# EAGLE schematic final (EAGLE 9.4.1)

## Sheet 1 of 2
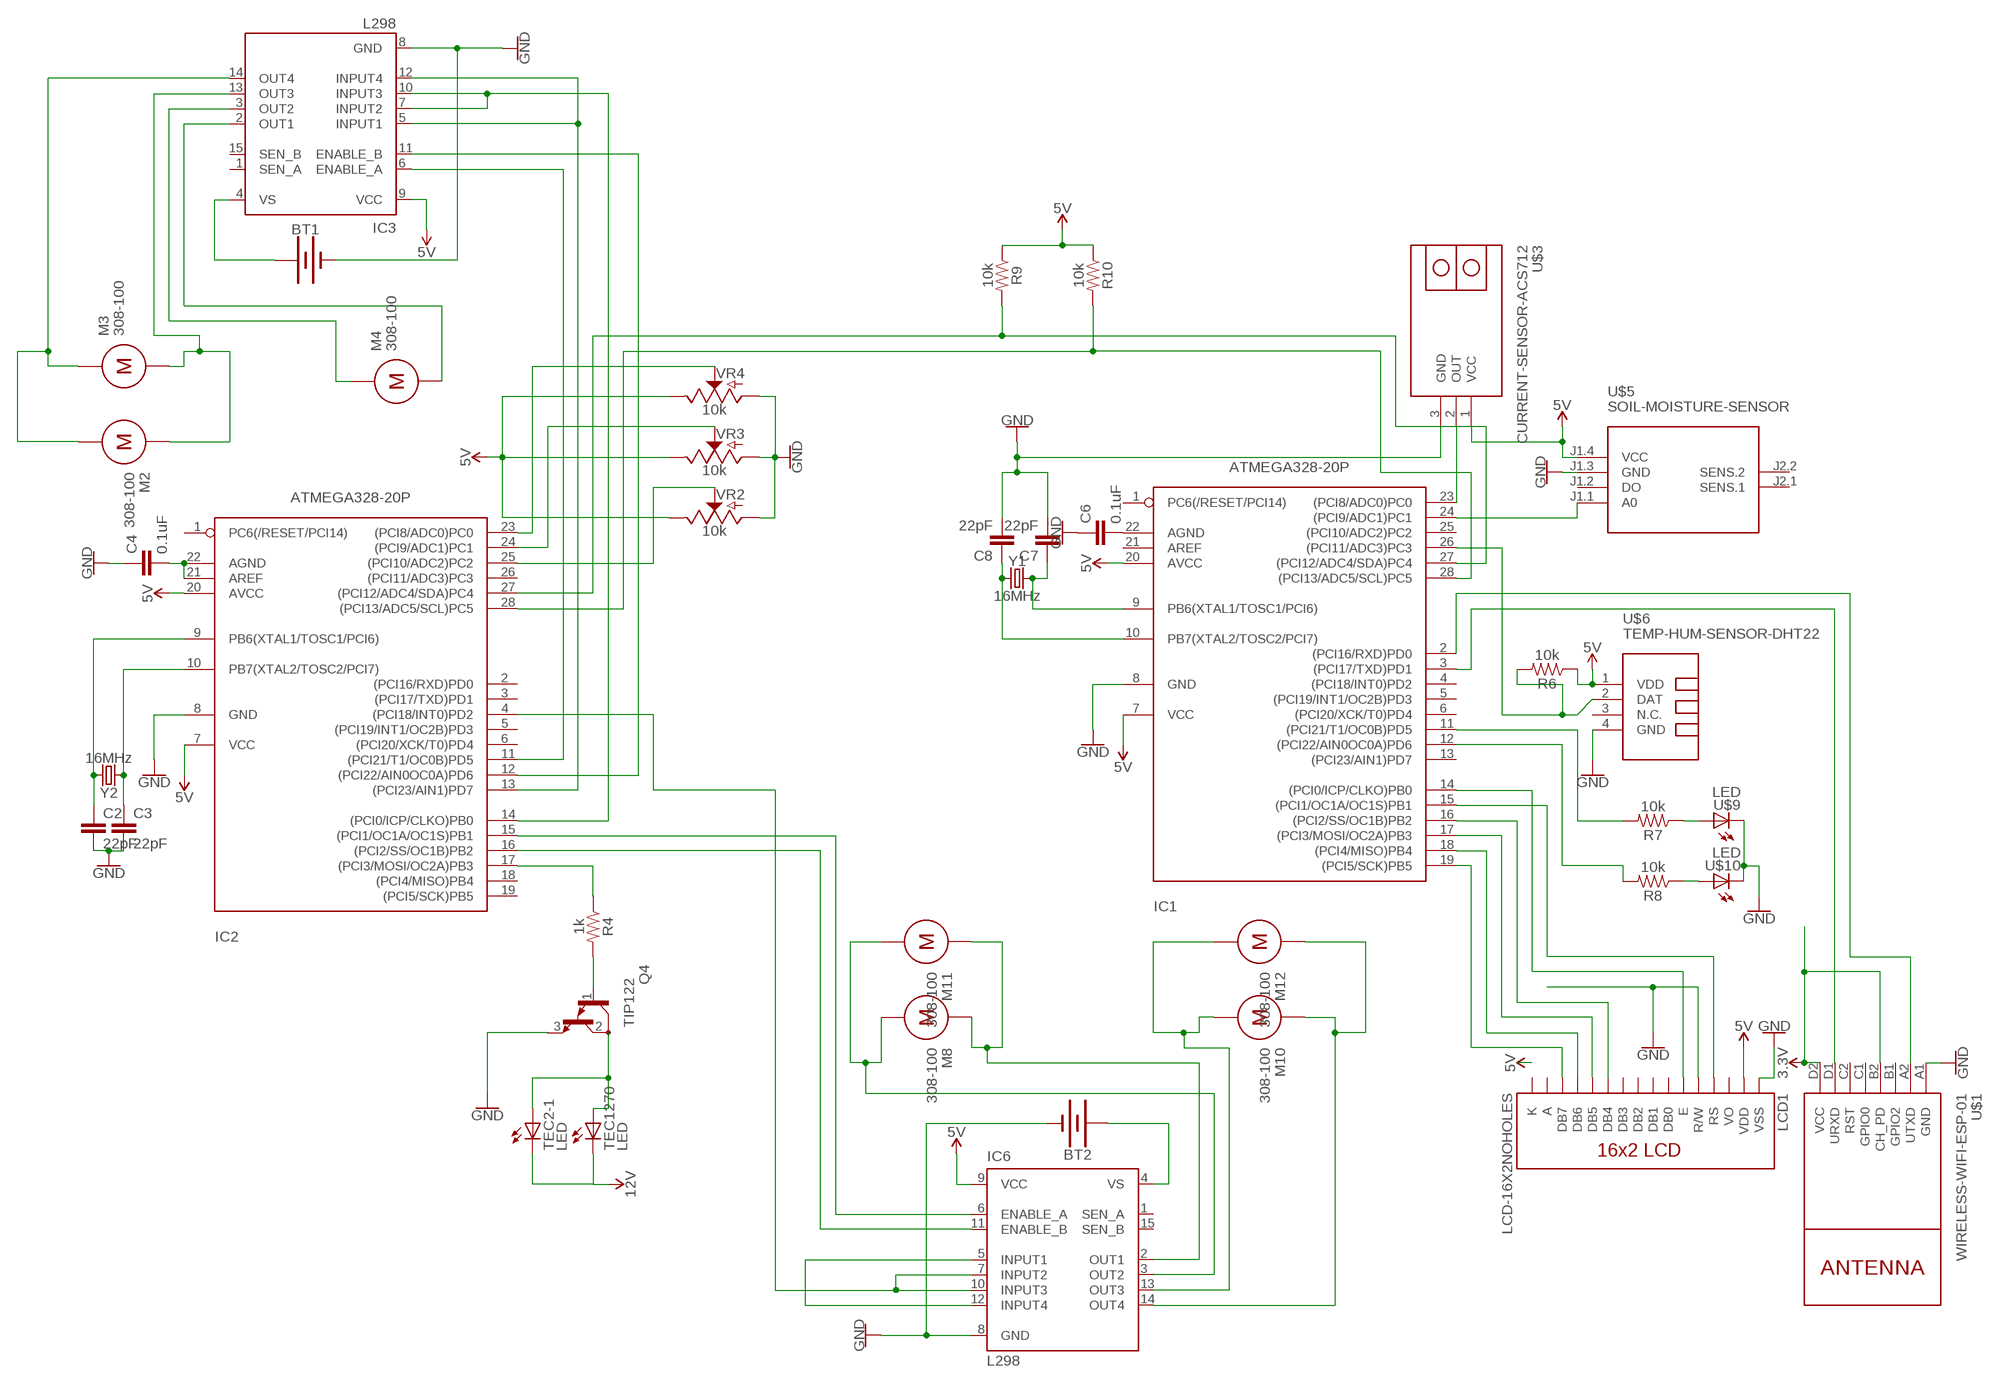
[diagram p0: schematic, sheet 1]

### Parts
BT1  BATTERY-12MM_PTH  [BATTCON_12MM_PTH]
BT2  BATTERY-12MM_PTH  [BATTCON_12MM_PTH]
C2  22pF  22PF-0603-50V-5%  [0603]
C3  22pF  22PF-0603-50V-5%  [0603]
C4  0.1uF  0.1UF-0402-16V-10%  [0402]
C6  0.1uF  0.1UF-0402-16V-10%  [0402]
C7  22pF  22PF-0603-50V-5%  [0603]
C8  22pF  22PF-0603-50V-5%  [0603]
IC1  ATMEGA328-20P  [DIL28-3]
IC2  ATMEGA328-20P  [DIL28-3]
IC3  L298  [MULTIWATT-15]
IC6  L298  [MULTIWATT-15]
LCD1  LCD-16X2NOHOLES  [LCD-16X2_NOHOLESNOSILK]
M2  308-100  [308-100]
M3  308-100  [308-100]
M4  308-100  [308-100]
M8  308-100  [308-100]
M10  308-100  [308-100]
M11  308-100  [308-100]
M12  308-100  [308-100]
Q4  TIP122  [TO220]
R4  1k  10KOHM-0603-1/10W-1%  [0603]
R6  10k  10KOHM-0603-1/10W-1%  [0603]
R7  10k  10KOHM-0603-1/10W-1%  [0603]
R8  10k  10KOHM-0603-1/10W-1%  [0603]
R9  10k  10KOHM-0603-1/10W-1%  [0603]
R10  10k  10KOHM-0603-1/10W-1%  [0603]
TEC2-1  LED  [HLMP-1790]
TEC1270  LED  [HLMP-1790]
U$1  WIRELESS-WIFI-ESP-01  [WIRELESS-WIFI-ESP-01]
U$3  CURRENT-SENSOR-ACS712  [CURRENT-SENSOR-ACS712]
U$5  SOIL-MOISTURE-SENSOR  [SOIL-MOISTURE-SENSOR]
U$6  TEMP-HUM-SENSOR-DHT22  [TEMP-HUM-SENSOR-DHT22]
U$9  LED  [HLMP-1790]
U$10  LED  [HLMP-1790]
VR2  10k  POTENTIOMETER-PTH-9MM-1/20W-20%-KIT  [POT-PTH-ALPS-KIT]
VR3  10k  POTENTIOMETER-PTH-9MM-1/20W-20%-KIT  [POT-PTH-ALPS-KIT]
VR4  10k  POTENTIOMETER-PTH-9MM-1/20W-20%-KIT  [POT-PTH-ALPS-KIT]
Y1  16MHz  CRYSTAL-16MHZPTH-HC49US  [HC49US]
Y2  16MHz  CRYSTAL-16MHZPTH-HC49US  [HC49US]

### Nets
3.3V: U$1.B2(CH_PD) U$1.D2(VCC) ; also sheet 2
5V: IC1.7(VCC) IC1.20(AVCC) IC2.7(VCC) IC2.20(AVCC) IC3.9(VCC) IC6.9(VCC) LCD1.2(VDD) R6.1 R9.1 R10.1 TEC2-1.C TEC1270.C U$3.1(VCC) U$5.J1.4(VCC) U$6.1(VDD) VR2.P$1(E) VR3.P$1(E) VR4.P$1(E) ; supply symbol labelled 12V ; also sheet 2
GND: BT1.GND(-) BT2.GND(-) C2.2 C3.2 C4.1 C6.1 C7.2 C8.2 IC1.8(GND) IC2.8(GND) IC3.8(GND) IC6.8(GND) LCD1.1(VSS) LCD1.5(R/W) Q4.3(E) U$1.A1(GND) U$3.3(GND) U$5.J1.3(GND) U$6.4(GND) U$9.C U$10.C VR2.P$3(A) VR3.P$3(A) VR4.P$3(A) ; also sheet 2
N$1: LCD1.14(DB7)
N$2: IC1.27((PCI12/ADC4/SDA)PC4) IC2.27((PCI12/ADC4/SDA)PC4) R9.2
N$3: IC2.25((PCI10/ADC2)PC2) VR2.P$2(S)
N$4: LCD1.13(DB6)
N$5: LCD1.12(DB5)
N$7: IC1.26((PCI11/ADC3)PC3) R6.2 U$6.2(DAT)
N$8: BT2.VCC@1(+) IC6.4(VS)
N$9: IC1.2((PCI16/RXD)PD0)
N$10: IC2.23((PCI8/ADC0)PC0) VR4.P$2(S)
N$11: C4.2 IC2.21(AREF) IC2.22(AGND)
N$14: IC1.23((PCI8/ADC0)PC0) U$3.2(OUT)
N$15: IC1.24((PCI9/ADC1)PC1) U$5.J1.1(A0)
N$16: IC1.19((PCI5/SCK)PB5)
N$17: IC1.18((PCI4/MISO)PB4)
N$18: IC1.17((PCI3/MOSI/OC2A)PB3)
N$19: IC6.5(INPUT1) IC6.12(INPUT4)
N$20: IC1.16((PCI2/SS/OC1B)PB2)
N$21: IC1.14((PCI0/ICP/CLKO)PB0)
N$22: IC1.15((PCI1/OC1A/OC1S)PB1)
N$23: IC2.4((PCI18/INT0)PD2) IC6.7(INPUT2) IC6.10(INPUT3)
N$24: IC2.12((PCI22/AIN0OC0A)PD6) IC3.11(ENABLE_B)
N$25: IC2.14((PCI0/ICP/CLKO)PB0) IC3.7(INPUT2) IC3.10(INPUT3)
N$26: IC3.2(OUT1) M4.NEG
N$29: BT1.VCC@1(+) IC3.4(VS)
N$30: IC2.11((PCI21/T1/OC0B)PD5) IC3.6(ENABLE_A)
N$31: IC2.15((PCI1/OC1A/OC1S)PB1) IC6.6(ENABLE_A)
N$32: IC2.16((PCI2/SS/OC1B)PB2) IC6.11(ENABLE_B)
N$33: IC6.2(OUT1) M8.POS M11.POS
N$34: IC3.3(OUT2) M4.POS
N$35: IC6.3(OUT2) M8.NEG M11.NEG
N$36: Q4.2(C) TEC2-1.A TEC1270.A
N$38: Q4.1(B) R4.2
N$39: LCD1.11(DB4)
N$40: LCD1.6(E)
N$41: IC2.24((PCI9/ADC1)PC1) VR3.P$2(S)
N$42: IC2.17((PCI3/MOSI/OC2A)PB3) R4.1
N$43: C3.1 IC2.10(PB7(XTAL2/TOSC2/PCI7)) Y2.1
N$44: IC2.13((PCI23/AIN1)PD7) IC3.5(INPUT1) IC3.12(INPUT4)
N$45: C2.1 IC2.9(PB6(XTAL1/TOSC1/PCI6)) Y2.2
N$46: IC1.3((PCI17/TXD)PD1)
N$47: IC1.11((PCI21/T1/OC0B)PD5) R7.2
N$48: IC1.12((PCI22/AIN0OC0A)PD6) R8.2
N$49: R7.1 U$9.A
N$50: R8.1 U$10.A
N$51: C6.2 IC1.22(AGND)
N$53: LCD1.4(RS)
N$54: U$1.A2(UTXD)
N$55: U$1.D1(URXD)
N$62: C8.1 IC1.10(PB7(XTAL2/TOSC2/PCI7)) Y1.1
N$63: C7.1 IC1.9(PB6(XTAL1/TOSC1/PCI6)) Y1.2
N$92: IC1.28((PCI13/ADC5/SCL)PC5) IC2.28((PCI13/ADC5/SCL)PC5) R10.2
O1: IC6.13(OUT3) M10.NEG M12.NEG
O2: IC6.14(OUT4) M10.POS M12.POS
O3: IC3.13(OUT3) M2.POS M3.NEG
O4: IC3.14(OUT4) M2.NEG M3.POS
Unconnected: IC1.1(PC6(/RESET/PCI14)) IC1.4((PCI18/INT0)PD2) IC1.5((PCI19/INT1/OC2B)PD3) IC1.6((PCI20/XCK/T0)PD4) IC1.13((PCI23/AIN1)PD7) IC1.21(AREF) IC1.25((PCI10/ADC2)PC2) IC2.1(PC6(/RESET/PCI14)) IC2.2((PCI16/RXD)PD0) IC2.3((PCI17/TXD)PD1) IC2.5((PCI19/INT1/OC2B)PD3) IC2.6((PCI20/XCK/T0)PD4) IC2.18((PCI4/MISO)PB4) IC2.19((PCI5/SCK)PB5) IC2.26((PCI11/ADC3)PC3) IC3.1(SEN_A) IC3.15(SEN_B) IC6.1(SEN_A) IC6.15(SEN_B) LCD1.3(VO) LCD1.7(DB0) LCD1.8(DB1) LCD1.9(DB2) LCD1.10(DB3) U$1.B1(GPIO2) U$1.C1(GPIO0) U$1.C2(RST) U$5.J1.2(DO) U$5.J2.1(SENS.1) U$5.J2.2(SENS.2) U$6.3(N.C.)

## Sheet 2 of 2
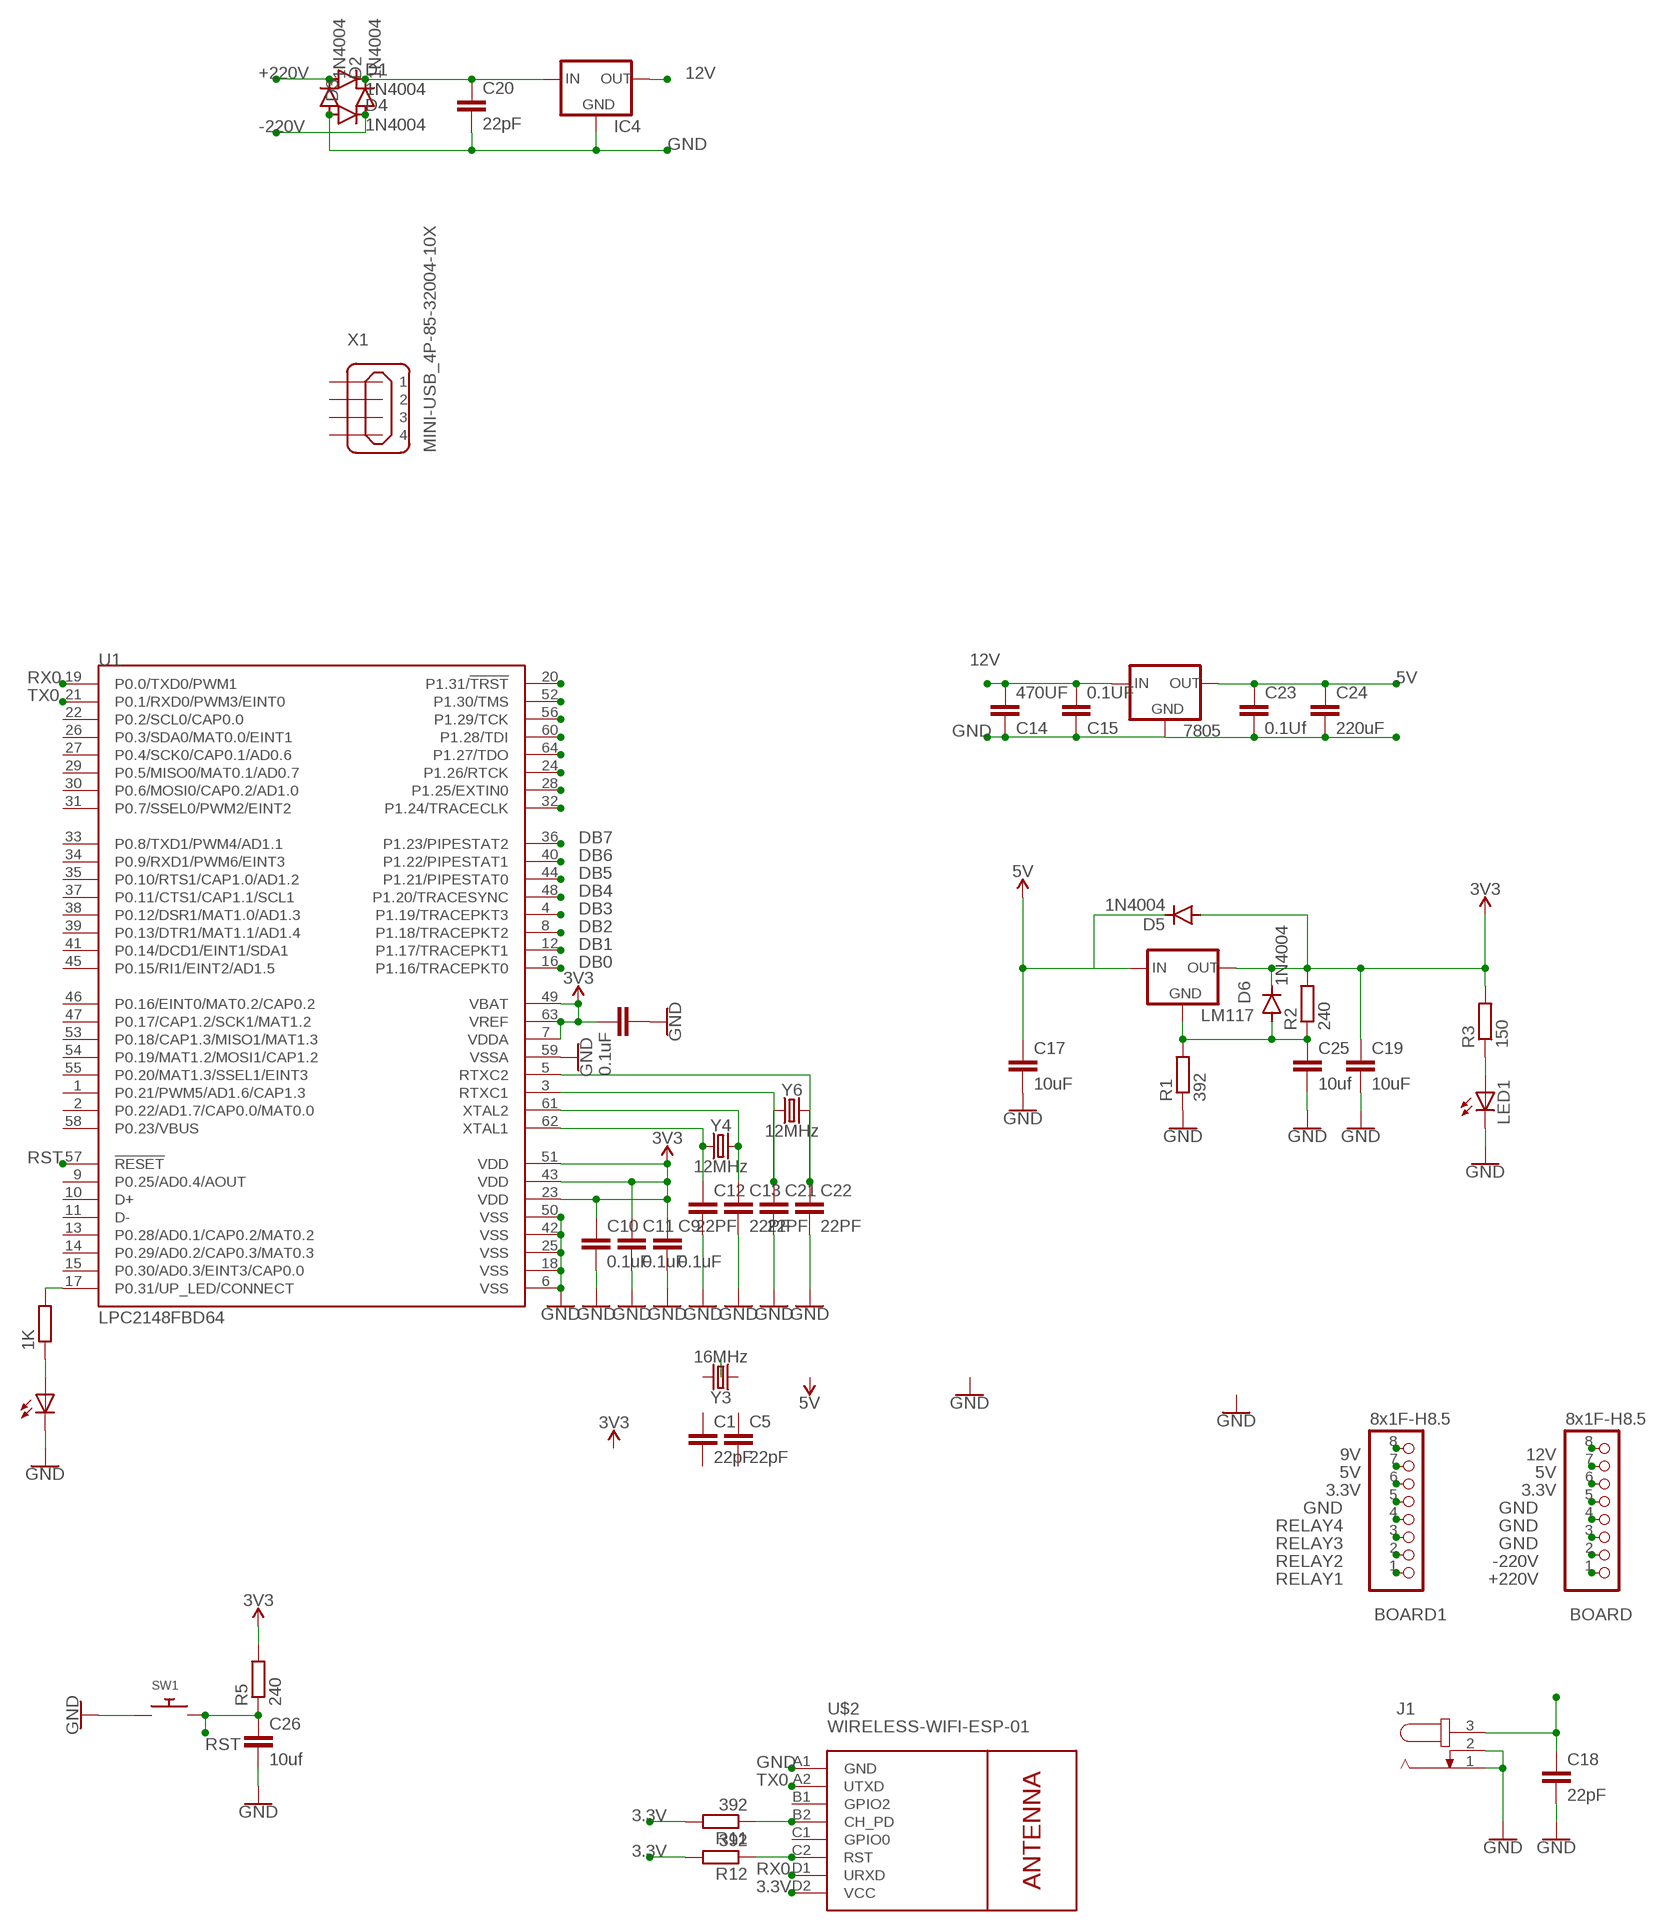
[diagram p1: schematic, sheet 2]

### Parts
1K  1k  R-EU_0204/5  [0204/5]
7805  78XXL  [78XXL]
BOARD  8x1F-H8.5  PINHD-1X8  [1X08]
BOARD1  8x1F-H8.5  PINHD-1X8  [1X08]
C1  22pF  22PF-0603-50V-5%  [0603]
C5  22pF  22PF-0603-50V-5%  [0603]
C9  0.1uF  22PF-0603-50V-5%  [0603]
C10  0.1uF  22PF-0603-50V-5%  [0603]
C11  0.1uF  22PF-0603-50V-5%  [0603]
C12  22PF  22PF-0603-50V-5%  [0603]
C13  22PF  22PF-0603-50V-5%  [0603]
C14  470UF  22PF-0603-50V-5%  [0603]
C15  0.1UF  22PF-0603-50V-5%  [0603]
C16  0.1uF  22PF-0603-50V-5%  [0603]
C17  10uF  22PF-0603-50V-5%  [0603]
C18  22pF  22PF-0603-50V-5%  [0603]
C19  10uF  22PF-0603-50V-5%  [0603]
C20  22pF  22PF-0603-50V-5%  [0603]
C21  22PF  22PF-0603-50V-5%  [0603]
C22  22PF  22PF-0603-50V-5%  [0603]
C23  0.1Uf  22PF-0603-50V-5%  [0603]
C24  220uF  22PF-0603-50V-5%  [0603]
C25  10uf  22PF-0603-50V-5%  [0603]
C26  10uf  22PF-0603-50V-5%  [0603]
D1  1N4004  [DO41-10]
D2  1N4004  [DO41-10]
D3  1N4004  [DO41-10]
D4  1N4004  [DO41-10]
D5  1N4004  [DO41-10]
D6  1N4004  [DO41-10]
IC4  78XXL  [78XXL]
J1  JACK-PLUG1  [SPC4078]
LED1  LED5MM  [LED5MM]
LED2  LED5MM  [LED5MM]
LM117  78XXL  [78XXL]
R1  392  R-EU_0204/5  [0204/5]
R2  240  R-EU_0204/5  [0204/5]
R3  150  R-EU_0204/5  [0204/5]
R5  240  R-EU_0204/5  [0204/5]
R11  392  R-EU_0204/5  [0204/5]
R12  392  R-EU_0204/5  [0204/5]
SW1  SWITCH_PUSHBUTTONC&K_KSS  [BTN_CK_KSS]
U1  LPC2148FBD64  [TSQFP50P1200X1200X160-64N]
U$2  WIRELESS-WIFI-ESP-01  [WIRELESS-WIFI-ESP-01]
X1  MINI-USB_4P-85-32004-10X  [85-32004-10X]
Y3  16MHz  CRYSTAL-16MHZPTH-HC49US  [HC49US]
Y4  12MHz  CRYSTAL-16MHZPTH-HC49US  [HC49US]
Y6  12MHz  CRYSTAL-16MHZPTH-HC49US  [HC49US]

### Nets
3.3V: BOARD1.6 BOARD.6 R11.2 R12.2 U$2.D2(VCC) ; also sheet 1
5V: 7805.OUT BOARD1.7 BOARD.7 C9.1 C10.1 C11.1 C16.2 C17.1 C19.1 C23.1 C24.1 D5.A D5.C D6.C LM117.IN LM117.OUT R2.2 R3.2 R5.2 U1.7(VDDA) U1.23(VDD) U1.43(VDD) U1.49(VBAT) U1.51(VDD) U1.63(VREF) ; supply symbol labelled 3V3 ; also sheet 1
9V: BOARD1.8
12V: 7805.IN BOARD.8 C14.1 C15.1 C18.1 IC4.OUT J1.3
+220V: BOARD.1 D1.A D3.C
-220V: BOARD.2 D2.A D4.C
DB0: U1.16(P1.16/TRACEPKT0)
DB1: U1.12(P1.17/TRACEPKT1)
DB2: U1.8(P1.18/TRACEPKT2)
DB3: U1.4(P1.19/TRACEPKT3)
DB4: U1.48(P1.20/TRACESYNC)
DB5: U1.44(P1.21/PIPESTAT0)
DB6: U1.40(P1.22/PIPESTAT1)
DB7: U1.36(P1.23/PIPESTAT2)
GND: 7805.GND BOARD1.5 BOARD.3 BOARD.4 BOARD.5 C9.2 C10.2 C11.2 C12.2 C13.2 C14.2 C15.2 C16.1 C17.2 C18.2 C19.2 C20.2 C21.2 C22.2 C23.2 C24.2 C25.2 C26.2 D3.A D4.A IC4.GND J1.1 J1.2 LED1.K(C) LED2.K(C) R1.1 SW1.P$1 U1.6(VSS) U1.18(VSS) U1.25(VSS) U1.42(VSS) U1.50(VSS) U1.59(VSSA) U$2.A1(GND) ; also sheet 1
N$6: C12.1 U1.62(XTAL1) Y4.1
N$12: C13.1 U1.61(XTAL2) Y4.2
N$28: C21.1 U1.3(RTXC1) Y6.1
N$37: C25.1 D6.A LM117.GND R1.2 R2.1
N$52: C22.1 U1.5(RTXC2) Y6.2
N$56: C20.1 D1.C D2.C IC4.IN
N$57: LED1.A R3.1
N$58: 1K.1 LED2.A
N$59: 1K.2 U1.17(P0.31/UP_LED/CONNECT)
N$66: U1.32(P1.24/TRACECLK)
N$67: U1.28(P1.25/EXTIN0)
N$68: U1.24(P1.26/RTCK)
N$69: U1.64(P1.27/TDO)
N$70: U1.60(P1.28/TDI)
N$71: U1.20(P1.31/!TRST)
N$72: U1.52(P1.30/TMS)
N$73: U1.56(P1.29/TCK)
N$74: R11.1 U$2.B2(CH_PD)
N$75: R12.1 U$2.C2(RST)
RELAY1: BOARD1.1
RELAY2: BOARD1.2
RELAY3: BOARD1.3
RELAY4: BOARD1.4
RST: C26.1 R5.1 SW1.P$2 U1.57(!RESET)
RX0: U1.19(P0.0/TXD0/PWM1) U$2.D1(URXD)
TX0: U1.21(P0.1/RXD0/PWM3/EINT0) U$2.A2(UTXD)
Unconnected: C1.1 C1.2 C5.1 C5.2 U1.1(P0.21/PWM5/AD1.6/CAP1.3) U1.2(P0.22/AD1.7/CAP0.0/MAT0.0) U1.9(P0.25/AD0.4/AOUT) U1.10(D+) U1.11(D-) U1.13(P0.28/AD0.1/CAP0.2/MAT0.2) U1.14(P0.29/AD0.2/CAP0.3/MAT0.3) U1.15(P0.30/AD0.3/EINT3/CAP0.0) U1.22(P0.2/SCL0/CAP0.0) U1.26(P0.3/SDA0/MAT0.0/EINT1) U1.27(P0.4/SCK0/CAP0.1/AD0.6) U1.29(P0.5/MISO0/MAT0.1/AD0.7) U1.30(P0.6/MOSI0/CAP0.2/AD1.0) U1.31(P0.7/SSEL0/PWM2/EINT2) U1.33(P0.8/TXD1/PWM4/AD1.1) U1.34(P0.9/RXD1/PWM6/EINT3) U1.35(P0.10/RTS1/CAP1.0/AD1.2) U1.37(P0.11/CTS1/CAP1.1/SCL1) U1.38(P0.12/DSR1/MAT1.0/AD1.3) U1.39(P0.13/DTR1/MAT1.1/AD1.4) U1.41(P0.14/DCD1/EINT1/SDA1) U1.45(P0.15/RI1/EINT2/AD1.5) U1.46(P0.16/EINT0/MAT0.2/CAP0.2) U1.47(P0.17/CAP1.2/SCK1/MAT1.2) U1.53(P0.18/CAP1.3/MISO1/MAT1.3) U1.54(P0.19/MAT1.2/MOSI1/CAP1.2) U1.55(P0.20/MAT1.3/SSEL1/EINT3) U1.58(P0.23/VBUS) U$2.B1(GPIO2) U$2.C1(GPIO0) X1.1 X1.2 X1.3 X1.4 Y3.1 Y3.2

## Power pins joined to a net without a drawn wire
A: LCD1.15(A)
K: LCD1.16(K)

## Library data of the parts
1K R1-R3 R5 R11 R12 = resistor:R-EU_: RESISTOR, European symbol
7805 IC4 LM117 = v-reg:78XXL: VOLTAGE REGULATOR
BOARD BOARD1 = SmartPrj:PINHD-1X8: PIN HEADER
BT1 BT2 = SparkFun-Batteries:BATTERY: Battery - Single Cell; PROD_ID: BATT-08315; SF_SKU: PRT-07948
C1-C3 C5 C7 C8 C18 C20 = SparkFun-Capacitors:22PF: 22pF ceramic capacitors; PROD_ID: CAP-07876
C4 C6 = SparkFun-Capacitors:0.1UF: 0.1µF ceramic capacitors; PROD_ID: CAP-12416
C9-C17 C19 C21-C26 = SparkFun-Capacitors:22PF: 22pF ceramic capacitors; PROD_ID: CAP-07876; VALUE: 22pF
D1-D6 = diode:1N4004: DIODE
IC1 IC2 = atmega328:ATMEGA328*P: MICROCONTROLLER 32 kBytes FLASH 2 kBytes SRAM 1 kBytes EEPROM USART 8-channel 10 bit ADC
IC3 IC6 = st-microelectronics-2:L298: DUAL FULL-BRIDGE DRIVER
J1 = con-jack:JACK-PLUG: DC POWER JACK Power Jack, DC, Right Angle, Through Hole, Rated 5A at 16VDC, PC Terminals Distributor: Farnell (www.Farnell.de) Drawing: 84N1161.pdf / 84N1162.pdf Manufacturer: SPC Technology (www.spctechnology.com) Type: SPC4077 / SPC 4078; OC_FARNELL: unknown; OC_NEWARK: unknown
LCD1 = SparkFun-Displays:LCD-16X2: Standard text-only 16x2 parallel input LCD Basic 16 character by 2 line display. Typically utilizes the extremely common HD44780 parallel interface chipset SparkFun Products: Basic 16x2 Green Basic 8x2 Green; SF_ID: LCD-00255
LED1 LED2 = adafruit:LED: LED
M2-M4 M8 M10-M12 = motor:308-100: Pico Vibe; PRECISION_MICRODRIVES: 308-100
Q4 = transistor-npn:TIP122*: NPN Darlington Transistor
R4 = SparkFun-Resistors:10KOHM: 10kΩ resistor; PROD_ID: RES-00824; VALUE: 10k
R6-R10 = SparkFun-Resistors:10KOHM: 10kΩ resistor; PROD_ID: RES-00824
SW1 = adafruit:SWITCH_PUSHBUTTON: Buttons
TEC2-1 TEC1270 U$9 U$10 = Ava:LED
U1 = philips-5:LPC2148
U$1 U$2 = diy-modules:WIRELESS-WIFI-ESP-01: Wireless Wi-Fi ESP-01 Module based on ESP8266 chip Click here to find device on ebay.com
U$3 = diy-modules:CURRENT-SENSOR-ACS712: Isolated Bipolar Current Sensors based on ACS712 chip More details available here: http://embedded-lab.com/blog/a-brief-overview-of-allegro-acs712-current-sensor-part-1/ Click here to find device on ebay.com Note: There are many available versions with different pinout. Please check before use
U$5 = diy-modules:SOIL-MOISTURE-SENSOR: Soil Moisture Sensor Click here to find device on ebay.com
U$6 = diy-modules:TEMP-HUM-SENSOR-DHT22: DHT22 - digital humidity & temperature sensor Also known as: AM2302 AM2302 datasheet available here: http://akizukidenshi.com/download/ds/aosong/AM2302.pdf Click here to find device on ebay.com
VR2-VR4 = SparkFun-Resistors:POTENTIOMETER: Potentiometer (Pot) Three-terminal potentiometers, with an adjustable wiper and two adjustable resistors. A pot can be used to create a configurable voltage divider, or as a variable resistor. Variants ALPS_POT and ALPS_POT_KIT - PTH, breadboard compatible, 9mm square pots Rotary Potentiometer -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; PROD_ID: RES-09177; SF_SKU: COM-09288
X1 = con-cypressindustries:MINI-USB_4P-: MINI USB 4 Pol. Source: www.cypressindustries.com
Y1-Y3 = SparkFun-Clocks:CRYSTAL-16MHZ: 16MHz Crystal; PROD_ID: XTAL-08181; SF_ID: COM-00536
Y4 Y6 = SparkFun-Clocks:CRYSTAL-16MHZ: 16MHz Crystal; PROD_ID: XTAL-08181; SF_ID: COM-00536; VALUE: 16MHz

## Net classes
0 default: width 1.016 mm, clearance 0.381 mm

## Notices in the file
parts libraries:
diy-modules: Released under the Creative Commons Attribution 4.0 International License: http://creativecommons.org/licenses/by/4.0
SparkFun-Capacitors: Licensing: Creative Commons ShareAlike 4.0 International - https://creativecommons.org/licenses/by-sa/4.0
philips-5: Copyright 2006 Weartronics
